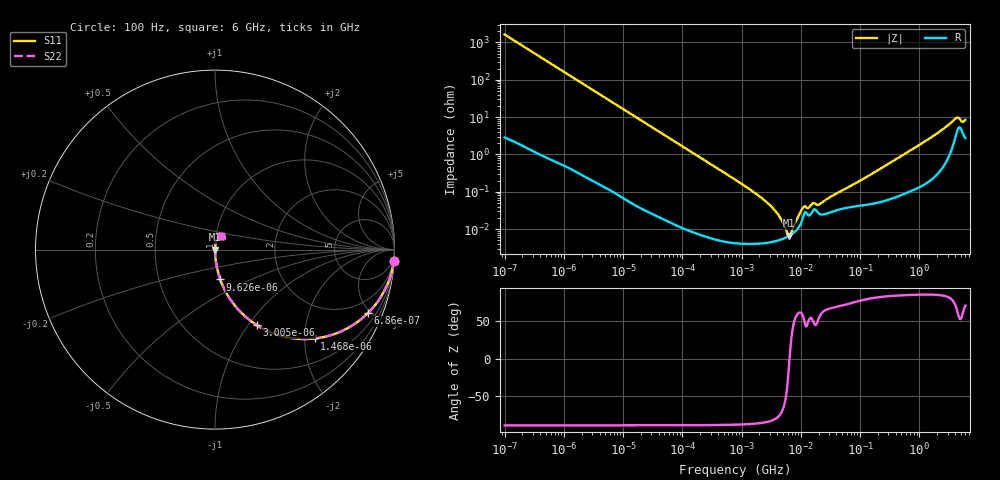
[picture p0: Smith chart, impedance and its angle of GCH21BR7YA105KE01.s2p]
!Murata Part Number: GCH21BR7YA105KE01
!These Parameters are Measured in Series Mode Connection
!Data Generated on Mar 13, 2026
!  o--ll--o
!Port1  Port2
!  o------o
!Operation Temp=25[degC], DC Bias Voltage=0[V]
!Freq. Start=100[Hz] Stop=6[GHz] 401[Steps]
# Hz S RI R 50
!Freq.(Hz) S11(Real) S11(Imag) S21(Real) S21(Imag) S12(Real) S12(Imag) S22(Real) S22(Imag)
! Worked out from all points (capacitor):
!   401 points, 100 Hz to 6 GHz, reference 50 ohm
!   read as one part in series: C = 973 nF near 109 Hz
!   lowest |Z| = 6.7 mohm at 6.353 MHz (marker M1)
!   series resonance near 6.462 MHz, so ESL is about 620 pH
!   S11 on the Smith chart (normalised r, x): 100 Hz: 1, -33; 686 Hz: 1.01, -4.78; 1.468 kHz: 1.01, -2.24; 3.005 kHz: 1.00, -1.09; 9.626 kHz: 1.00, -0.34; 6 GHz: 1.05, +0.16
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100  0.9962 -0.0609  0.00383 0.0609  0.00383 0.0609  0.9962 -0.0609
335  0.9594 -0.1961  0.0406 0.1961  0.0406 0.1961  0.9594 -0.1961
686  0.8504 -0.3553  0.1496 0.3553  0.1496 0.3553  0.8504 -0.3553
1468  0.5556 -0.4953  0.4444 0.4953  0.4444 0.4953  0.5556 -0.4953
2008  0.4013 -0.4885  0.5987 0.4885  0.5987 0.4885  0.4013 -0.4885
3005  0.2313 -0.4199  0.7687 0.4199  0.7687 0.4199  0.2313 -0.4199
5143  0.0939 -0.2898  0.9061 0.2898  0.9061 0.2898  0.0939 -0.2898
9626  0.0292 -0.1663  0.9708 0.1663  0.9708 0.1663  0.0292 -0.1663
40335  0.00189 -0.041  0.9981 0.041  0.9981 0.041  0.00189 -0.041
774597  4.63e-05 -0.00212  1 0.00212  1 0.00212  4.63e-05 -0.00212
2837864  4.35e-05 -0.000476  1 0.000476  1 0.000476  4.35e-05 -0.000476
4060267  4.91e-05 -0.000251  1 0.000251  1 0.000251  4.91e-05 -0.000251
5554849  5.93e-05 -7.97e-05  0.9999 7.97e-05  0.9999 7.97e-05  5.93e-05 -7.97e-05
6353432  6.64e-05 -8.9e-06  0.9999 8.9e-06  0.9999 8.9e-06  6.64e-05 -8.9e-06
7599586  8.08e-05 8.8e-05  0.9999 -8.8e-05  0.9999 -8.8e-05  8.08e-05 8.8e-05
1.087309e7  0.000202 0.000315  0.9998 -0.000315  0.9998 -0.000315  0.000202 0.000315
1.555665e7  0.000286 0.000379  0.9997 -0.000379  0.9997 -0.000379  0.000286 0.000379
2.128304e7  0.00025 0.000402  0.9998 -0.000402  0.9998 -0.000402  0.00025 0.000402
3.124326e8  0.000654 0.00576  0.9993 -0.00576  0.9993 -0.00576  0.000654 0.00576
1.712697e9  0.00325 0.0309  0.9968 -0.0309  0.9968 -0.0309  0.00325 0.0309
4.009986e9  0.0323 0.08  0.9677 -0.08  0.9677 -0.08  0.0323 0.08
6e9  0.0326 0.0753  0.9674 -0.0753  0.9674 -0.0753  0.0326 0.0753
